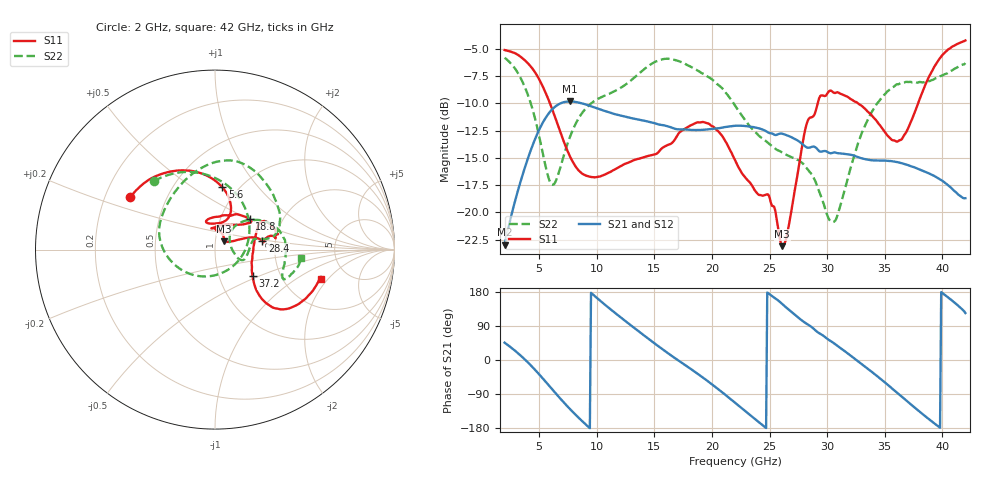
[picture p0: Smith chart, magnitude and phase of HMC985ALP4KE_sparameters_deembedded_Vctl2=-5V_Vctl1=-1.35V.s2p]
!s2p File: Measurements: S11, S21, S12, S22
# GHz S dB R 50.0
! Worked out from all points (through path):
!   401 points, 2 GHz to 42 GHz, reference 50 ohm
!   highest |S21| = -9.84 dB at 7.7 GHz (marker M1); lowest = -23.0 dB at 2 GHz (marker M2)
!   lowest |S11| = -23.1 dB at 26.1 GHz (marker M3), VSWR 1.15, Z = 55.2 + j5.21 ohm
!   |S11| at or under -10 dB: 5.935 GHz to 29.18 GHz (23.24 GHz wide, 132 % of centre); 32.66 GHz to 37.9 GHz (5.235 GHz wide, 14.8 % of centre)
!   |S22| runs from -20.9 to -5.8 dB; largest |S21 - S12| = 0.00033
!   S11 on the Smith chart (normalised r, x): 2 GHz: 0.31, +0.26; 5.6 GHz: 0.84, +0.67; 18.8 GHz: 1.37, +0.50; 28.4 GHz: 1.71, +0.18; 37.2 GHz: 1.45, -0.45; 42 GHz: 3.23, -1.68
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2  -5.12 148.1  -22.98 45.7  -22.98 45.7  -5.83 131.8
3.6  -5.92 121.6  -16.43 5.9  -16.43 5.9  -8.14 87.6
4.7  -7.26 100.6  -13.14 -27.8  -13.14 -27.8  -11.64 45.7
5.6  -9.14 83.2  -11.27 -58.6  -11.28 -58.6  -15.97 -8.6
6.3  -11.04 72.6  -10.39 -83.3  -10.39 -83.3  -17.41 -70.3
7.7  -14.93 68.5  -9.84 -130.3  -9.84 -130.3  -13.01 -151.7
8.7  -16.42 79.3  -10.01 -160.4  -10.01 -160.4  -10.93 -178.5
10.1  -16.75 96.6  -10.49 161.4  -10.50 161.5  -9.60 159.9
12  -15.81 107.9  -11.12 114.3  -11.12 114.3  -8.64 135.2
15.4  -14.43 80.4  -11.96 35.3  -11.96 35.4  -6.06 84.8
18.8  -11.74 41.5  -12.45 -37.4  -12.46 -37.4  -7.02 43.4
22  -15.21 52.8  -12.07 -112.7  -12.07 -112.7  -10.19 11.9
24.9  -18.38 94.4  -12.69 175.8  -12.70 175.8  -13.66 10.4
26.1  -23.10 42.2  -12.79 147.8  -12.80 147.8  -14.52 -2.3
28.4  -11.42 10.5  -14.08 92.4  -14.09 92.4  -16.19 -21.7
28.7  -11.26 8.7  -13.99 85.8  -13.99 85.8  -16.57 -21.5
30.6  -9.05 15.2  -14.51 43.8  -14.51 43.8  -20.86 21.7
33.2  -10.43 31.1  -15.10 -15.5  -15.11 -15.5  -12.26 42.2
35.4  -13.13 8.7  -15.29 -69.1  -15.29 -69.0  -8.78 19.2
37.2  -11.87 -34.9  -15.74 -115.3  -15.74 -115.3  -8.04 -1.1
39.7  -6.00 -41.6  -16.90 -176.4  -16.90 -176.4  -7.61 -23.5
42  -4.24 -15.4  -18.70 123.9  -18.71 124.0  -6.32 -5.9
